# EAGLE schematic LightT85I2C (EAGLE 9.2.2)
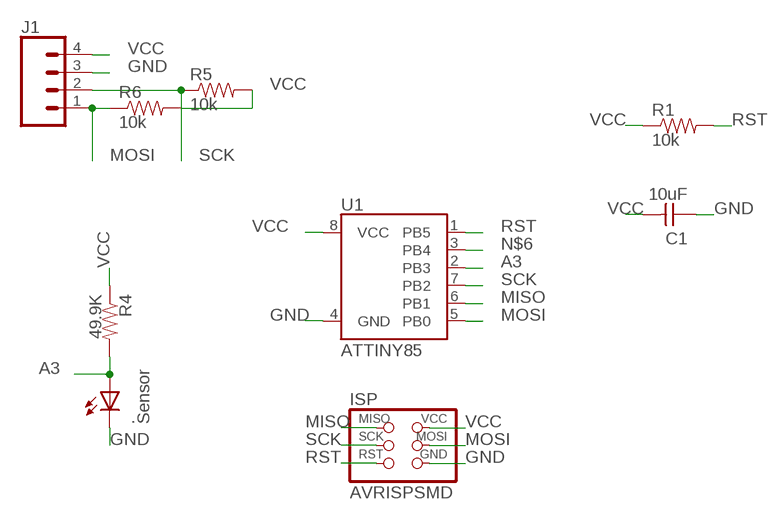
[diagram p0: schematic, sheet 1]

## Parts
.  Sensor  LEDFAB1206  [LED1206FAB]
C1  10uF  CAP-UNPOLARIZEDFAB  [C1206FAB]
ISP  AVRISPSMD  [2X03SMD]
J1  CONN_04SMD_RA_FEMALE  [1X04_SMD_RA_FEMALE]
R1  10k  RESISTOR1206  [1206]
R4  49.9K  RESISTOR1206  [1206]
R5  10k  RESISTOR1206  [1206]
R6  10k  RESISTOR1206  [1206]
U1  ATTINY85  [ATTINY85]

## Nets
A3: ..1(A) R4.2 U1.2(PB3)
GND: ..2(C) C1.1 ISP.6(GND) J1.3 U1.4(GND)
MISO: ISP.1(MISO) U1.6(PB1)
MOSI: ISP.4(MOSI) J1.1 R6.1 U1.5(PB0)
N$6: U1.3(PB4)
RST: ISP.5(RST) R1.2 U1.1(PB5)
SCK: ISP.3(SCK) J1.2 R5.1 U1.7(PB2)
VCC: C1.2 ISP.2(VCC) J1.4 R1.1 R4.1 R5.2 R6.2 U1.8(VCC)

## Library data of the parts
. = fab:LED: LED
C1 = fab:CAP-UNPOLARIZED
ISP = fab:AVRISP
J1 = SparkFun-Connectors:CONN_04: Multi connection point. Often used as Generic Header-pin footprint for 0.1 inch spaced/style header connections On any of the 0.1 inch spaced packages, you can populate with these: Break Away Headers - Straight (PRT-00116) Break Away Male Headers - Right Angle (PRT-00553) Female Headers (PRT-00115)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; PROD_ID: CONN-12382
R1 R4-R6 = SparkFun-Resistors:RESISTOR: Generic Resistor Package
U1 = SparkFun-IC-Microcontroller:ATTINY85; PROD_ID: IC-09092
